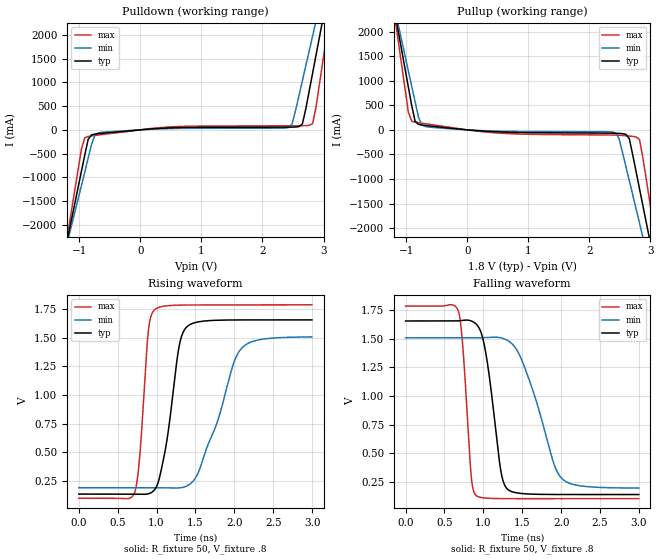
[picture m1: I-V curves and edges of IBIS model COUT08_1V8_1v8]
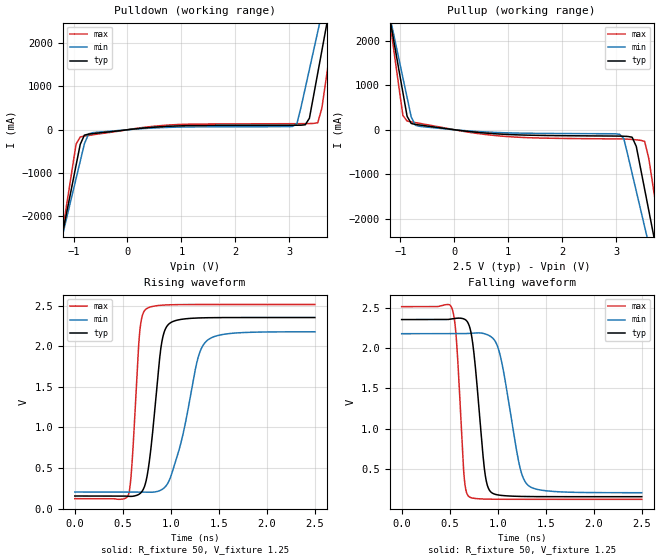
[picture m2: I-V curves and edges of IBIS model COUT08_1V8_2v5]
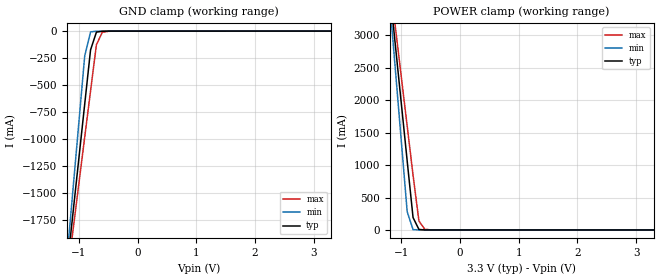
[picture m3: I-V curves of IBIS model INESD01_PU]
|   This file is an IBIS representation of the   |
|   Integrated Device Technology, Inc.   |
|   ICS8312   |
[IBIS Ver]   4.1
[File name]   8312_3v3vdd.ibs
[File Rev]   0.0
[Date]   20 Mar 2009 | Last modified
|   May 18 2006 | Generated
[Source]   Originated at Integrated Devices Technology, Inc.
[Disclaimer]
IDT hereby grants the user of this IBIS model a non-exclusive,
nontransferable license to use this IBIS model under the following terms.
Before using this IBIS model, the user should read this license.
If the user does not accept these terms,  the IBIS model should be
returned to IDT within 30 days.
   The user is granted this license only to use the IBIS model and
is not granted rights to sell, load, rent, lease or license the IBIS
model in whole or in part, or in modified form to anyone other than
user. User may modify the IBIS model to suit its specific
applications but rights to derivative works and such modifications
shall belong to IDT.
   This IBIS model is provided on an "AS IS" basis and IDT makes
absolutely no warranty with respect to the information contained
herein. IDT DISCLAIMS AND CUSTOMER WAIVES ALL WARRANTIES, EXPRESS
OR IMPLIED, INCLUDING WARRANTIES OF MERCHANTABILITY OR FITNESS FOR
A PARTICULAR PURPOSE. The entire risk as to quality and performance
is with the Customer. ACCORDINGLY, IN NO EVENT SHALL THE COMPANY BE
LIABLE FOR ANY DAMAGES, WHETHER IN CONTRACT OR TORT,INCLUDING ANY
LOST PROFITS OR OTHER INCIDENTAL, CONSEQUENTIAL, EXEMPLARY, OR
PUNITIVE DAMAGES ARISING OUT OF THE USE OR APPLICATION OF THE IBIS
model provided in this package. Further, IDT reserves the right to
make changes without notice to any product herein to improve
reliability, function, or design. IDT does not convey any license
under patent rights or any other intellectual property rights,
including those of third parties.
   IDT is not obligated to provide maintenance or support
for the licensed IBIS model.
[Copyright]   Copyright 2006 by Integrated Device Technology, Inc.
[Component]   ICS8312AY_3v3VDD
[Manufacturer] Integrated Devices Technology, Inc.
[Package]
|LQFP32
|lead + wire   typ   min   max
R_pkg   220.4m   212.5m   238m
L_pkg   1.841n   1.708n   1.974n
C_pkg   0.316p   0.2907p   0.33p
[Pin] signal_name   model_name   R_pin   L_pin   C_pin
1   GND   GND   238m   1.974n   0.330p
2   VDD   POWER   225m   1.841n   0.311p
3   CLK_EN   INESD01_PU   218m   1.7745n   0.301p
4   CLK   INESD01_PD   213m   1.708n   0.291p
5   GND   GND   213m   1.708n   0.291p
6   OE   INESD01_PU   218m   1.7745n   0.301p
7   VDD   POWER   225m   1.841n   0.311p
8   GND   GND   238m   1.974n   0.330p
9   Q11   COUT08_1V8   238m   1.974n   0.330p
10   VDDO   POWER   225m   1.841n   0.311p
11   Q10   COUT08_1V8   218m   1.7745n   0.301p
12   GND   GND   213m   1.708n   0.291p
13   Q9   COUT08_1V8   213m   1.708n   0.291p
14   VDDO   POWER   218m   1.7745n   0.301p
15   Q8   COUT08_1V8   225m   1.841n   0.311p
16   GND   GND   238m   1.974n   0.330p
17   GND   GND   238m   1.974n   0.330p
18   Q7   COUT08_1V8   225m   1.841n   0.311p
19   VDDO   POWER   218m   1.7745n   0.301p
20   Q6   COUT08_1V8   213m   1.708n   0.291p
21   GND   GND   213m   1.708n   0.291p
22   Q5   COUT08_1V8   218m   1.7745n   0.301p
23   VDDO   POWER   225m   1.841n   0.311p
24   Q4   COUT08_1V8   238m   1.974n   0.330p
25   GND   GND   238m   1.974n   0.330p
26   Q3   COUT08_1V8   225m   1.841n   0.311p
27   VDDO   POWER   218m   1.7745n   0.301p
28   Q2   COUT08_1V8   213m   1.708n   0.291p
29   GND   GND   213m   1.708n   0.291p
30   Q1   COUT08_1V8   218m   1.7745n   0.301p
31   VDDO   POWER   225m   1.841n   0.311p
32   Q0   COUT08_1V8   238m   1.974n   0.330p
[Model Selector] COUT08_1V8
COUT08_1V8_1v8  Buffer selection for VDD=3.3 and VDDO=1v8
COUT08_1V8_2v5  Buffer selection for VDD=3.3 and VDDO=2v5
COUT08_1V8_3v3  Buffer selection for VDD=3.3 and VDDO=3v3
| Models and submodels in the file (5): COUT08_1V8_1v8 (Output), COUT08_1V8_2v5 (Output), INESD01_PU (Input), INESD01_PD (Input), COUT08_1V8_3v3 (Output)
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[Model] COUT08_1V8_1v8
Model_type   Output
Polarity   Non-Inverting
Vmeas = .9
Rref = 50
Cref = 0
Vref = .9
|   typ   min   max
C_comp   2pF   1.5pF   2.5pF
|   typ   min   max
[Voltage range]  1.8V   1.710V   1.890V
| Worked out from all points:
|   slope of the pulldown table from 0 to 0.27 V, typ, clamps not added: 9.88 ohm
|   slope of the pullup table from 0 to 0.27 V, typ, clamps not added: 10.2 ohm
|   rising waveform, R_fixture 50, V_fixture .8: 20-80 % time 183ps typ, 371ps min, 99.6ps max; typ from 0.136 V to 1.66 V
|   falling waveform, R_fixture 50, V_fixture .8: 20-80 % time 167ps typ, 350ps min, 94.1ps max; typ from 1.66 V to 0.136 V
[pulldown]
|Voltage   I (typ)   I (min)   I (max)
-1.8V     -6.086A    -5.51A     -7.053A
-1.188V   -2.264A    -2.328A    -2.18A
-964.9mV  -872.6mA   -1.171A    -403.1mA
-797.9mV  -105.5mA   -304.5mA   -128mA
-630.9mV  -73.03mA   -52.89mA   -98.95mA
2.431V    57.5mA     51.11mA    84.22mA
2.487V    58.15mA    128.3mA    84.46mA
2.654V    127.4mA    1.037A     87.27mA
2.821V    1.195A     1.976A     131.6mA
2.988V    2.325A     2.916A     1.44A
3.099V    3.08A      3.544A     2.406A
3.6V      6.485A     6.374A     6.76A
[pullup]
|Voltage   I (typ)   I (min)   I (max)
-1.8V     6.59A      5.952A     7.666A
-1.188V   2.402A     2.47A      2.315A
-1.132V   2.021A     2.154A     1.828A
-909.3mV  497.2mA    887.8mA    177.3mA
-686.6mV  89.4mA     66.76mA    124.8mA
2.431V    -69.97mA   -64.65mA   -107.2mA
2.654V    -178.5mA   -1.033A    -126.6mA
2.765V    -850.9mA   -1.607A    -143.7mA
2.821V    -1.197A    -1.895A    -198mA
2.932V    -1.889A    -2.47A     -1.01A
3.099V    -2.928A    -3.334A    -2.338A
3.6V      -6.049A    -5.931A    -6.322A
[Ramp]
|   typ   min   max
dV/dt_r   1.218/0.277n   1.055/0.523n   1.354/0.153n
dV/dt_f   1.222/0.25n   1.057/0.51n   1.359/0.139n
[Rising Waveform]
R_fixture = 50
V_fixture = .8
V_fixture_max = .945
V_fixture_min = .855
C_fixture = 0.0p
| Time   typ   min   max
0s        136.4mV    192.4mV    100.1mV
716.1ps   136mV      192.4mV    144.4mV
784.3ps   134.6mV    192.5mV    467.2mV
895.9ps   138.9mV    192.6mV    1.566V
979.6ps   178.6mV    192.1mV    1.748V
1.122ns   557.9mV    190.4mV    1.779V
1.293ns   1.434V     190.3mV    1.786V
1.383ns   1.591V     204.9mV    1.787V
2.086ns   1.656V     1.403V     1.787V
2.998ns   1.657V     1.508V     1.79V
[Falling Waveform]
R_fixture = 50
V_fixture = .8
V_fixture_max = .945
V_fixture_min = .855
C_fixture = 0.0p
| Time   typ   min   max
0s        1.657V     1.509V     1.787V
675.8ps   1.658V     1.509V     1.748V
734.7ps   1.663V     1.509V     1.438V
843.2ps   1.658V     1.509V     298.4mV
908.3ps   1.629V     1.51V      127mV
1.02ns    1.418V     1.511V     105.9mV
1.218ns   369.5mV    1.51V      100.8mV
1.305ns   186.6mV    1.488V     100.4mV
1.999ns   136.7mV    284.1mV    100.1mV
2.998ns   136.5mV    193.1mV    100.4mV
[Model] COUT08_1V8_2v5
Model_type   Output
Polarity   Non-Inverting
Vmeas = 1.25
Rref = 50
Cref = 0
Vref = 1.25
|   typ   min   max
C_comp   2pF   1.5pF   2.5pF
|   typ   min   max
[Voltage range]  2.5V   2.375V   2.625V
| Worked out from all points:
|   slope of the pulldown table from 0 to 0.375 V, typ, clamps not added: 7.84 ohm
|   slope of the pullup table from 0 to 0.375 V, typ, clamps not added: 7.16 ohm
|   rising waveform, R_fixture 50, V_fixture 1.25: 20-80 % time 112ps typ, 213ps min, 68ps max; typ from 0.154 V to 2.35 V
|   falling waveform, R_fixture 50, V_fixture 1.25: 20-80 % time 98.3ps typ, 168ps min, 64.8ps max; typ from 2.35 V to 0.154 V
[pulldown]
|Voltage   I (typ)   I (min)   I (max)
-2.5V     -10.49A    -9.183A    -12.66A
-1.186V   -2.276A    -2.339A    -2.192A
-953.6mV  -822.7mA   -1.13A     -335.8mA
-876.3mV  -338.3mA   -728mA     -166.6mA
-721.6mV  -101.9mA   -96.8mA    -132.4mA
3.067V    103.7mA    77.59mA    139.5mA
3.144V    104.2mA    145mA      139.8mA
3.376V    267mA      1.397A     142.7mA
3.531V    1.311A     2.267A     161.1mA
3.686V    2.358A     3.138A     1.175A
3.84V     3.408A     4.011A     2.517A
5V        11.31A     10.58A     12.63A
[pullup]
|Voltage   I (typ)   I (min)   I (max)
-2.5V     11.44A     9.986A     13.84A
-1.186V   2.424A     2.488A     2.34A
-953.6mV  831.7mA    1.165A     319.1mA
-876.3mV  301.5mA    723.9mA    195.5mA
-721.6mV  119.6mA    100.8mA    160.4mA
3.067V    -143.2mA   -101.8mA   -206.5mA
3.144V    -146.2mA   -200mA     -208.2mA
3.299V    -167.8mA   -983.4mA   -218.7mA
3.531V    -1.337A    -2.181A    -261.5mA
3.686V    -2.299A    -2.981A    -1.261A
3.84V     -3.261A    -3.781A    -2.49A
5V        -10.49A    -9.798A    -11.71A
[Ramp]
|   typ   min   max
dV/dt_r   1.764/0.173n   1.582/0.32n   1.921/0.103n
dV/dt_f   1.774/0.148n   1.589/0.253n   1.936/0.098n
[Rising Waveform]
R_fixture = 50
V_fixture = 1.25
V_fixture_max = 1.3125
V_fixture_min = 1.1875
C_fixture = 0.0p
| Time   typ   min   max
0s        154.1mV    203.2mV    121.3mV
557.2ps   150.3mV    203.4mV    162.6mV
594.9ps   149.8mV    203.5mV    536.4mV
675.2ps   180.6mV    203.1mV    2.165V
743ps     342.6mV    201.5mV    2.459V
898.6ps   1.995V     228.1mV    2.506V
976.4ps   2.271V     328.8mV    2.511V
1.28ns    2.349V     1.844V     2.515V
1.365ns   2.352V     2.057V     2.515V
2.5ns     2.355V     2.179V     2.515V
[Falling Waveform]
R_fixture = 50
V_fixture = 1.25
V_fixture_max = 1.3125
V_fixture_min = 1.1875
C_fixture = 0.0p
| Time   typ   min   max
0s        2.355V     2.179V     2.515V
524.6ps   2.363V     2.179V     2.491V
572.3ps   2.371V     2.179V     2.069V
650.1ps   2.361V     2.179V     408.4mV
700.3ps   2.288V     2.184V     155.6mV
865.9ps   458.9mV    2.178V     124.6mV
928.7ps   212.3mV    2.143V     122.9mV
1.027ns   171.6mV    1.907V     121.8mV
1.308ns   156mV      306.2mV    121.3mV
2.5ns     154.1mV    203.3mV    121.3mV
[Model] INESD01_PU
Model_type   Input
Polarity   Non-Inverting
Vinl = 0.8V
Vinh = 2.0V
|   typ   min   max
C_comp   2pF   1.5pF   2.5pF
|   typ   min   max
[Voltage range]  3.3V   3.15V   3.45V
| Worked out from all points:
|   GND clamp passes 1 mA (typ) near -0.55 V on its own axis
|   POWER clamp passes 1 mA (typ) near -0.61 V on its own axis
[GND_clamp]
|Voltage   I(typ)   I(min)   I(max)
-3.3V     -12.83A    -15.14A    -11.37A
-1.2V     -2.195A    -2.092A    -2.281A
-1.1V     -1.689A    -1.472A    -1.849A
-900mV    -678.5mA   -232.7mA   -984.8mA
-800mV    -174mA     -7.237mA   -553.3mA
-700mV    -9.767mA   -1.114mA   -126.1mA
-600mV    -1.7mA     -240.1uA   -11.15mA
-300mV    -81.66uA   -67.79uA   -163.4uA
3.3V      1.866nA    1.113pA    239.1nA
[POWER_clamp]
|Voltage   I(typ)   I(min)   I(max)
-3.3V     22.38A     26.45A     19.82A
-1.2V     3.723A     3.545A     3.874A
-1.1V     2.836A     2.457A     3.116A
-1V       1.949A     1.369A     2.358A
-900mV    1.063A     281mA      1.601A
-800mV    191.5mA    5.012mA    843.9mA
-700mV    8.032mA    142.2uA    138.3mA
-600mV    607uA      17.63uA    10.62mA
-400mV    16.32uA    7.545uA    335.9uA
3.3V      -71.13uA   -62.11uA   -78.26uA
